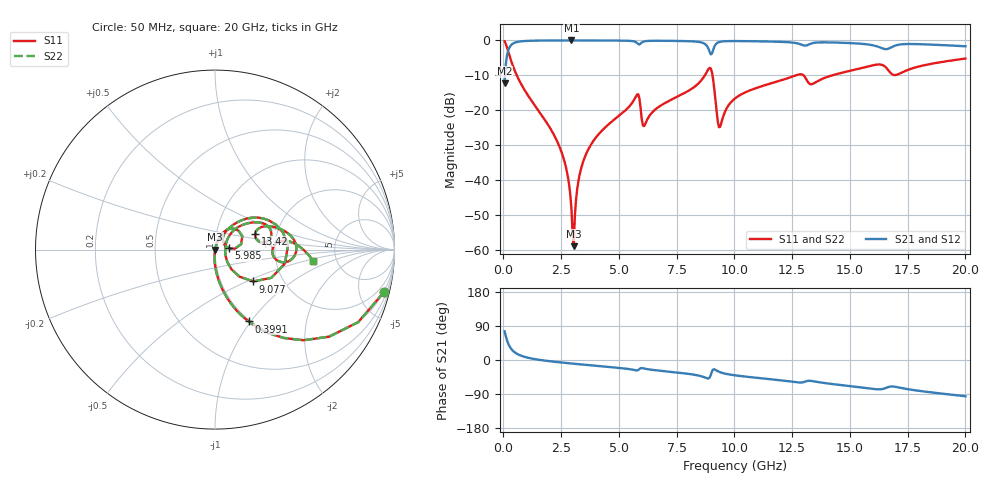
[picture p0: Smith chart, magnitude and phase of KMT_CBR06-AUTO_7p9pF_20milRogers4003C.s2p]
! Data measured by Modelithics Inc. support@modelithics.com 813-866-6335
! KEMET CBR06-AUTO 7.9pF, Pad Width= 0.851mm, Pad Length= 0.64mm, Pad Gap= 0.62mm, 20mil Rogers 4003C substrate Data, January 2022
# hz S ma R 50
! 2 Port Network Data from SP1.SP block
! freq  magS11  angS11  magS21  angS21  magS12  angS12  magS22  angS22
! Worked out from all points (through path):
!   401 points, 50 MHz to 20 GHz, reference 50 ohm
!   highest |S21| = -0.01 dB at 2.943 GHz (marker M1); lowest = -12.3 dB at 50 MHz (marker M2)
!   group delay of S21, straight-line fit = 14.5 ps
!   lowest |S11| = -58.8 dB at 3.042 GHz (marker M3), VSWR 1.00, Z = 50.1 + j0.0556 ohm
!   |S11| at or under -10 dB: 578.9 MHz to 8.719 GHz (8.14 GHz wide, 175 % of centre); 9.049 GHz to 12.65 GHz (3.604 GHz wide, 33.2 % of centre); 12.99 GHz to 14.23 GHz (1.234 GHz wide, 9.07 % of centre)
!   |S22| runs from -58.8 to -0.3 dB; largest |S21 - S12| = 0
!   S11 on the Smith chart (normalised r, x): 50 MHz: 0.98, -7.91; 399.1 MHz: 0.98, -0.97; 5.985 GHz: 1.16, +0.02; 9.077 GHz: 1.42, -0.55; 13.42 GHz: 1.55, +0.29; 20 GHz: 3.33, -0.60
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5e7  0.9701 -14.2  0.2426 75.8  0.2426 75.8  0.9701 -14.2
3.99125e8  0.4417 -65.0  0.8965 24.9  0.8965 24.9  0.4417 -65.0
2.444e9  0.02927 -94.6  0.9987 -6.2  0.9987 -6.2  0.02927 -94.6
2.74325e9  0.01351 -94.5  0.999 -8.1  0.999 -8.1  0.01351 -94.5
2.94275e9  0.003976 -86.5  0.999 -9.3  0.999 -9.3  0.003976 -86.5
3.0425e9  0.001145 29.0  0.999 -9.9  0.999 -9.9  0.001145 29.0
3.391625e9  0.01601 74.8  0.9988 -11.8  0.9988 -11.8  0.01601 74.8
3.990125e9  0.0404 73.3  0.9979 -15.2  0.9979 -15.2  0.0404 73.3
5.73575e9  0.1582 47.2  0.9455 -27.2  0.9455 -27.2  0.1582 47.2
5.985125e9  0.07646 6.0  0.9312 -21.2  0.9312 -21.2  0.07646 6.0
6.13475e9  0.06353 45.4  0.9747 -23.1  0.9747 -23.1  0.06353 45.4
6.73325e9  0.1129 59.5  0.9886 -28.1  0.9886 -28.1  0.1129 59.5
8.678375e9  0.3012 36.2  0.9085 -45.1  0.9085 -45.1  0.3012 36.2
8.92775e9  0.4064 2.8  0.6859 -46.5  0.6859 -46.5  0.4064 2.8
9.077375e9  0.2775 -39.7  0.7289 -24.9  0.7289 -24.9  0.2775 -39.7
9.376625e9  0.05789 9.4  0.9556 -32.1  0.9556 -32.1  0.05789 9.4
1.0025e10  0.148 45.8  0.979 -40.4  0.979 -40.4  0.148 45.8
1.276812e10  0.3252 22.7  0.9004 -59.2  0.9004 -59.2  0.3252 22.7
1.336662e10  0.2376 19.7  0.9122 -55.6  0.9122 -55.6  0.2376 19.7
1.34165e10  0.2416 21.7  0.92 -56.1  0.92 -56.1  0.2416 21.7
1.670825e10  0.3591 -10.3  0.7714 -70.6  0.7714 -70.6  0.3591 -10.3
2e10  0.5505 -6.6  0.8249 -95.7  0.8249 -95.7  0.5505 -6.6
